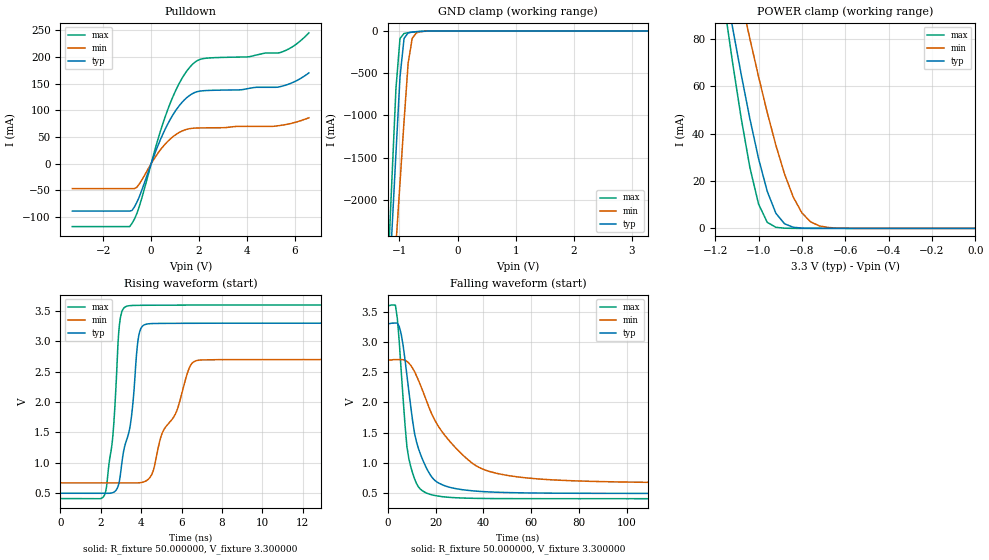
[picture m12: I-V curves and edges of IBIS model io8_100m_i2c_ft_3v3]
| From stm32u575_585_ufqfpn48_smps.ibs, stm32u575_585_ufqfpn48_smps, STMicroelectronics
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|   Model io8_100m_i2c_ft_3v3
[Model]  io8_100m_i2c_ft_3v3
Model_type I/O_open_drain
Polarity   Non-Inverting
Enable   Active-Low
Vinl =   0.990000V
Vinh =   2.310000V
Vmeas =  1.650000V
Cref =   50.000000pF
Rref =   100.000000M
Vref =   1.650000V
C_comp   3.320400pF   3.288500pF   3.361100pF
[Temperature Range]   25.000000   0.140000k   -40.000000
[Pullup Reference]   3.300000V   2.700000V   3.600000V
[Pulldown Reference]   0.0V   0.0V   0.0V
[POWER Clamp Reference]   3.300000V   2.700000V   3.600000V
[GND Clamp Reference]   0.0V   0.0V   0.0V
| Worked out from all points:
|   slope of the pulldown table from 0 to 0.495 V, typ, clamps not added: 8.84 ohm
|   GND clamp passes 1 mA (typ) near -0.51 V on its own axis
|   POWER clamp passes 1 mA (typ) near -0.85 V on its own axis
|   rising waveform, R_fixture 50.000000, V_fixture 3.300000: 20-80 % time 691ps typ, 1.39ns min, 418ps max; typ from 0.496 V to 3.3 V
|   falling waveform, R_fixture 50.000000, V_fixture 3.300000: 20-80 % time 7.46ns typ, 19.4ns min, 4.08ns max; typ from 3.3 V to 0.496 V
[Pulldown]
|Voltage   I(typ)   I(min)   I(max)
-3.3V     -88.61mA   -46.48mA   -117.6mA
-900mV    -88.61mA   -46.48mA   -117.6mA
-700mV    -80.76mA   -46.48mA   -103.5mA
-500mV    -62.15mA   -38.24mA   -80.45mA
300mV     35.76mA    20.75mA    48.11mA
800mV     83.04mA    46.39mA    113.4mA
1.3V      115.2mA    61.33mA    160.4mA
1.8V      132.8mA    66.57mA    188.9mA
2.3V      136.9mA    67.16mA    197.4mA
5.4V      144.2mA    71.57mA    207.9mA
6V        153.5mA    77.1mA     221.4mA
6.6V      169.9mA    86mA       244.9mA
[GND_clamp]
|Voltage   I(typ)   I(min)   I(max)
-3.3V     -9.848A    -9.957A    -9.458A
-1.2V     -3.312A    -4.013A    -2.863A
-1.13V    -2.381A    -3.274A    -1.769A
-1.06V    -1.452A    -2.535A    -684.7mA
-990mV    -542.9mA   -1.798A    -88.02mA
-920mV    -87.11mA   -1.064A    -28.44mA
-850mV    -22.1mA    -382.4mA   -19.61mA
-780mV    -11.97mA   -86.98mA   -13.71mA
-710mV    -7.619mA   -22.26mA   -8.745mA
-640mV    -4.493mA   -7.773mA   -4.817mA
-360mV    -31.22uA   -172.6uA   -8.607uA
3.28V     0A         15.66nA    -5.841nA
[POWER_clamp]
|Voltage   I(typ)   I(min)   I(max)
-3.28V    1.355A     1.167A     1.664A
-1.16V    105.7mA    131.6mA    95.69mA
-1.12V    84.97mA    114mA      70.27mA
-1.08V    65.05mA    96.83mA    46.54mA
-1.04V    46.34mA    80.15mA    25.76mA
-1V       29.51mA    64.13mA    10.3mA
-960mV    15.69mA    48.99mA    2.571mA
-920mV    6.373mA    35.1mA     455.6uA
-840mV    490.7uA    13.24mA    11.36uA
-760mV    27.33uA    2.767mA    276.6nA
-640mV    346.6nA    134.1uA    15.62nA
0V        0A         19.91nA    0A
[Ramp]
| variable   typ   min   max
dV/dt_r  1.68256/0.76960n   1.21961/1.44556n   1.91499/0.52845n
dV/dt_f  1.68256/7.44460n   1.21961/19.36115n   1.91499/4.06747n
R_load = 50.000000
[Rising Waveform]
R_fixture= 50.000000
V_fixture= 3.300000
V_fixture_min= 2.700000
V_fixture_max= 3.600000
|time   V(typ)   V(min)   V(max)
0s        495.7mV    667.3mV    408.3mV
2.202ns   495.5mV    667.2mV    483mV
2.603ns   507.1mV    666.9mV    1.467V
2.923ns   698.7mV    666.6mV    3.277V
3.243ns   1.34V      666.4mV    3.574V
3.524ns   1.776V     666.5mV    3.59V
3.844ns   3.022V     667.5mV    3.593V
4.164ns   3.273V     687.5mV    3.594V
6.727ns   3.298V     2.681V     3.598V
19.94ns   3.3V       2.7V       3.6V
[Falling Waveform]
R_fixture= 50.000000
V_fixture= 3.300000
V_fixture_min= 2.700000
V_fixture_max= 3.600000
|time   V(typ)   V(min)   V(max)
0s        3.3V       2.7V       3.6V
3.203ns   3.309V     2.706V     3.603V
5.606ns   3.127V     2.706V     2.516V
8.008ns   2.444V     2.676V     1.265V
9.61ns    1.928V     2.61V      936mV
12.81ns   1.239V     2.365V     603.4mV
19.22ns   728.5mV    1.739V     464.3mV
37.64ns   531.5mV    936.2mV    413.4mV
64.06ns   501.2mV    731.7mV    408.7mV
398.8ns   495.7mV    667.3mV    408.3mV
